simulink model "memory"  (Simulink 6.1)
settings: Solver=ode45  StartTime=0.0  StopTime=25.0  RelTol=1e-3
undefined symbols (not defined in the file or in its folder): memory_netlist
libraries: xbsIndex_r3 x12, adlibrary2 x2

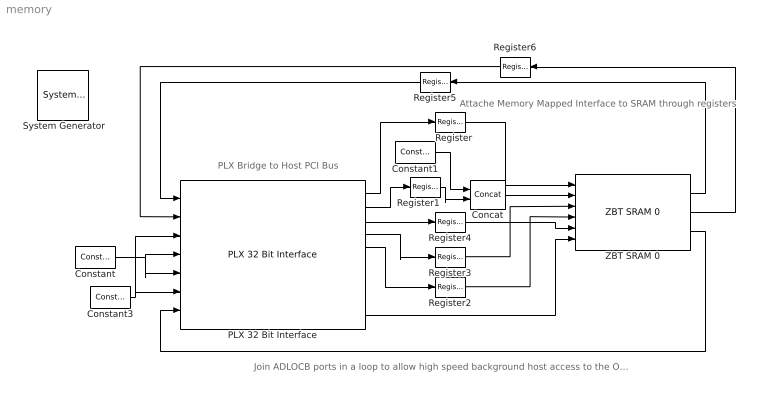
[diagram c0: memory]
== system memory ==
  note: PLX Bridge to Host PCI Bus
  note: Attache Memory Mapped Interface to SRAM through registers
  note: Join ADLOCB ports in a loop to allow high speed background host access to the Off Chip Ram
  " System Generator" : xbsIndex_r3/ System Generator  Tag=genX  xilinxfamily=Virtex2  part=xc2v4000  speed=-4  package=ff1152  synthesis_tool=XST  directory=./memory_netlist  testbench=off  simulink_period=1  sysclk_period=10  incr_netlist=off  trim_vbits=Everywhere in SubSystem  dbl_ovrd=According to Block Masks  core_generation=According to Block Masks  run_coregen=off  deprecated_control=off  eval_field=0
  Concat : xbsIndex_r3/Concat  num_inputs=2  explicit_period=off  period=1  dbl_ovrd=off
  Constant : xbsIndex_r3/Constant  const=0  equ=P=C  arith_type=Boolean  n_bits=1  bin_pt=0  opselect=C  inp2=PCIN>>17  opr=+  inp1=P  carry=CIN  iostate=0  explicit_period=on  period=1  dbl_ovrd=off
  Constant1 : xbsIndex_r3/Constant  const=0  equ=P=C  arith_type=Unsigned  n_bits=4  bin_pt=0  opselect=C  inp2=PCIN>>17  opr=+  inp1=P  carry=CIN  iostate=0  explicit_period=on  period=1  dbl_ovrd=off
  Constant3 : xbsIndex_r3/Constant  const=0  equ=P=C  arith_type=Unsigned  n_bits=32  bin_pt=0  opselect=C  inp2=PCIN>>17  opr=+  inp1=P  carry=CIN  iostate=0  explicit_period=on  period=1  dbl_ovrd=off
  PLX 32 Bit Interface : adlibrary2/ADM-XRC-II/PLX 32 Bit Interface  program='slave_write 0x0000 0xabcd1234;slave_read 0x0000'  clock_ratio=1.5
  Register{,1..4} (5 alike) : xbsIndex_r3/Register  init=0  reg_only_valid=off  explicit_period=on  period=1  rst=off  en=off  out_en=off  dbl_ovrd=off  show_param=off
  Register5 : xbsIndex_r3/Register  Orientation=left  init=0  reg_only_valid=off  explicit_period=on  period=1  rst=off  en=off  out_en=off  dbl_ovrd=off  show_param=off
  Register6 : xbsIndex_r3/Register  Orientation=left  init=0  reg_only_valid=off  explicit_period=on  period=1  rst=off  en=off  out_en=off  dbl_ovrd=off  show_param=off
  ZBT SRAM 0 : adlibrary2/ADM-XRC-II/ZBT SRAM 0
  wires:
  Constant/1 -> PLX 32 Bit Interface/4, PLX 32 Bit Interface/5
  Constant3/1 -> PLX 32 Bit Interface/6, PLX 32 Bit Interface/3
  PLX 32 Bit Interface/3 -> Register4/1
  PLX 32 Bit Interface/5 -> Register2/1
  PLX 32 Bit Interface/4 -> Register3/1
  PLX 32 Bit Interface/2 -> Register1/1
  PLX 32 Bit Interface/1 -> Register/1
  PLX 32 Bit Interface/10 -> ZBT SRAM 0/6
  ZBT SRAM 0/3 -> PLX 32 Bit Interface/7
  ZBT SRAM 0/2 -> Register6/1
  ZBT SRAM 0/1 -> Register5/1
  Register/1 -> ZBT SRAM 0/1
  Register2/1 -> ZBT SRAM 0/4
  Register3/1 -> ZBT SRAM 0/3
  Register4/1 -> ZBT SRAM 0/5
  Concat/1 -> ZBT SRAM 0/2
  Constant1/1 -> Concat/1
  Register1/1 -> Concat/2
  Register5/1 -> PLX 32 Bit Interface/1
  Register6/1 -> PLX 32 Bit Interface/2
